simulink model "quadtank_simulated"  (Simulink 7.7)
settings: Solver=ode45  StartTime=0.0  StopTime=150  FixedStep=0.01  RelTol=1e-6
PreLoadFcn:
  | init_quadtank
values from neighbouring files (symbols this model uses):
  Aaw = tf([1 2 1],[1])    [init_quadtank.m]
  C1 = 1/(s+1)    [init_quadtank.m]
  C2 = 1/(s+1)    [init_quadtank.m]
  W1 = eye(2)    [init_quadtank.m]
  W2 = eye(2)    [init_quadtank.m]
libraries: cstblocks x4, tank x1

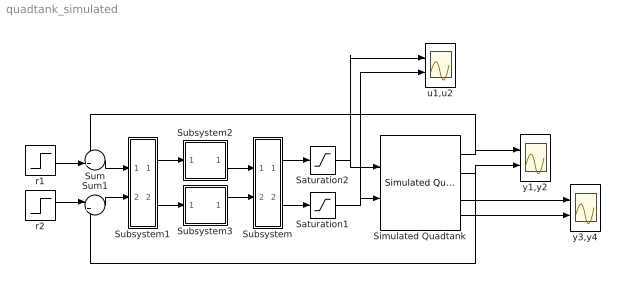
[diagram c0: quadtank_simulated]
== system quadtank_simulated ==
  Saturation1 : Saturate  UpperLimit=10  LowerLimit=0
  Saturation2 : Saturate  UpperLimit=10  LowerLimit=0
  Simulated Quadtank : tank/Simulated Quadtank  SystemSampleTime=-1  gamma1=0.7  gamma2=0.7
  Subsystem : Subsystem
  Subsystem1 : Subsystem
  Subsystem2 : Subsystem  mask(Controller C1){aw=off}
      mask prompts: aw "Antiwindup"
      mask help: Uses the LTI variable C1 from the workspace
  Subsystem3 : Subsystem  mask(Controller C2){aw=off}
      mask prompts: aw "Antiwindup"
      mask help: Uses the LTI variable C2 from the workspace
  Sum : Sum  Inputs=-+|
  Sum1 : Sum  Inputs=|+-
  r1 : Step  Time=50  Before=5  After=6  SampleTime=0
  r2 : Step  Time=100  Before=5  After=6  SampleTime=0
  u1,u2 : Scope  NumInputPorts=2
  y1,y2 : Scope  NumInputPorts=2
  y3,y4 : Scope  NumInputPorts=2
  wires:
  Simulated Quadtank/1 -> y1,y2/1, Sum/1
  Simulated Quadtank/2 -> y1,y2/2, Sum1/2
  r2/1 -> Sum1/1
  Simulated Quadtank/3 -> y3,y4/1
  Simulated Quadtank/4 -> y3,y4/2
  Saturation2/1 -> u1,u2/1, Simulated Quadtank/1
  Saturation1/1 -> u1,u2/2, Simulated Quadtank/2
  Subsystem2/1(u) -> Subsystem/1(In1)
  Subsystem3/1(u) -> Subsystem/2(In2)
  Subsystem1/1(Out1) -> Subsystem2/1(e)
  Subsystem1/2(Out2) -> Subsystem3/1(e)
  Subsystem/1(Out1) -> Saturation2/1
  Subsystem/2(Out2) -> Saturation1/1
  Sum/1 -> Subsystem1/1(In1)
  Sum1/1 -> Subsystem1/2(In2)
  r1/1 -> Sum/2

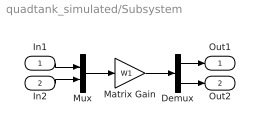
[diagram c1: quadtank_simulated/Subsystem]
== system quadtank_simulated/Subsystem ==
  In1 : Inport
  In2 : Inport  Port=2
  Demux : Demux  Outputs=2
  Matrix Gain : Gain  Gain=W1  Multiplication=Matrix(K*u)
  Mux : Mux  Inputs=2
  Out1 : Outport
  Out2 : Outport  Port=2
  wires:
  Demux/1 -> Out1/1
  In1/1 -> Mux/1
  Demux/2 -> Out2/1
  In2/1 -> Mux/2
  Mux/1 -> Matrix Gain/1
  Matrix Gain/1 -> Demux/1

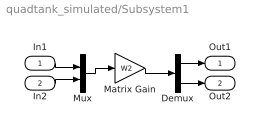
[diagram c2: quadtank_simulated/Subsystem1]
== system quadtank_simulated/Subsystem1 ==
  In1 : Inport
  In2 : Inport  Port=2
  Demux : Demux  Outputs=2
  Matrix Gain : Gain  Gain=W2  Multiplication=Matrix(K*u)
  Mux : Mux  Inputs=2
  Out1 : Outport
  Out2 : Outport  Port=2
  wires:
  Matrix Gain/1 -> Demux/1
  Mux/1 -> Matrix Gain/1
  In2/1 -> Mux/2
  Demux/2 -> Out2/1
  In1/1 -> Mux/1
  Demux/1 -> Out1/1

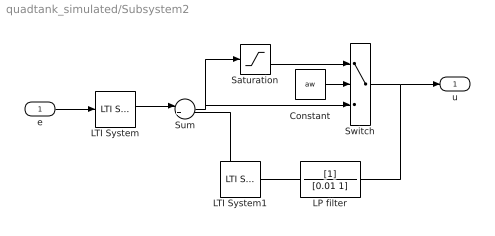
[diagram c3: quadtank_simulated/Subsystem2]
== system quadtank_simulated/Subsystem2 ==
  e : Inport
  Constant : Constant  Value=aw
  LP filter : TransferFcn  Denominator=[0.01 1]
  LTI System : cstblocks/LTI System  SystemSampleTime=-1  sys=tf(C1.num{:},1)/Aaw  IC=[]
  LTI System1 : cstblocks/LTI System  SystemSampleTime=-1  sys=(Aaw-tf(C1.den{:},1))/Aaw  IC=[]
  Saturation : Saturate  UpperLimit=10  LowerLimit=0
  Sum : Sum  Inputs=|++
  Switch : Switch  Threshold=0.5
  u : Outport
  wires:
  e/1 -> LTI System/1
  LTI System/1 -> Sum/1
  LTI System1/1 -> Sum/2
  Constant/1 -> Switch/2
  Switch/1 -> u/1, LP filter/1
  Saturation/1 -> Switch/1
  Sum/1 -> Switch/3, Saturation/1
  LP filter/1 -> LTI System1/1

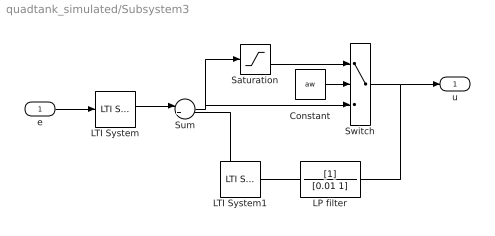
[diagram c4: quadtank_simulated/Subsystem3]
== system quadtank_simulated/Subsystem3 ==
  e : Inport
  Constant : Constant  Value=aw
  LP filter : TransferFcn  Denominator=[0.01 1]
  LTI System : cstblocks/LTI System  SystemSampleTime=-1  sys=tf(C2.num{:},1)/Aaw  IC=[]
  LTI System1 : cstblocks/LTI System  SystemSampleTime=-1  sys=(Aaw-tf(C2.den{:},1))/Aaw  IC=[]
  Saturation : Saturate  UpperLimit=10  LowerLimit=0
  Sum : Sum  Inputs=|++
  Switch : Switch  Threshold=0.5
  u : Outport
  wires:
  LP filter/1 -> LTI System1/1
  Sum/1 -> Saturation/1, Switch/3
  Saturation/1 -> Switch/1
  Switch/1 -> LP filter/1, u/1
  Constant/1 -> Switch/2
  LTI System1/1 -> Sum/2
  LTI System/1 -> Sum/1
  e/1 -> LTI System/1
